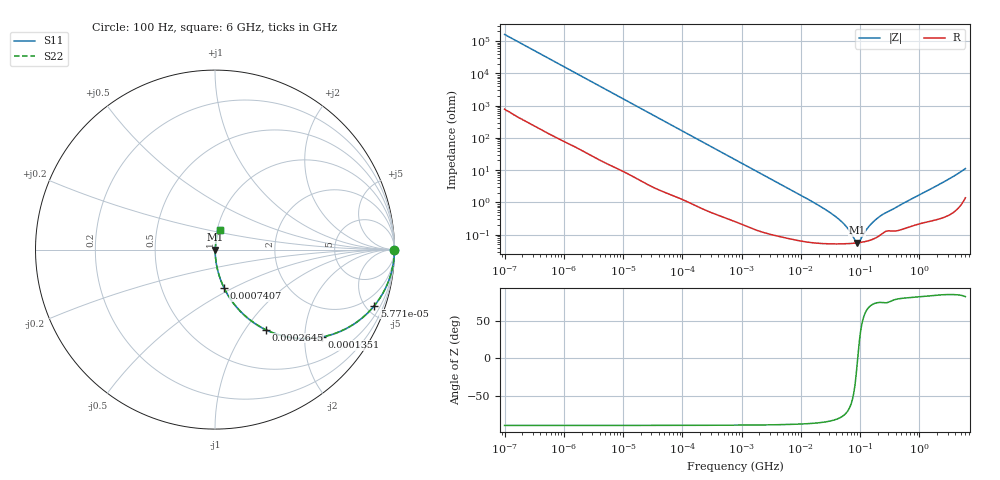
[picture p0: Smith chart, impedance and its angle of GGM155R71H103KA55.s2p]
!Murata Part Number: GGM155R71H103KA55
!These Parameters are Measured in Series Mode Connection
!Data Generated on Jun 19, 2026
!  o--ll--o
!Port1  Port2
!  o------o
!Operation Temp=25[degC], DC Bias Voltage=0[V]
!Freq. Start=100[Hz] Stop=6[GHz] 401[Steps]
# Hz S RI R 50
!Freq.(Hz) S11(Real) S11(Imag) S21(Real) S21(Imag) S12(Real) S12(Imag) S22(Real) S22(Imag)
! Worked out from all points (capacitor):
!   401 points, 100 Hz to 6 GHz, reference 50 ohm
!   read as one part in series: C = 9.88 nF near 109 Hz
!   lowest |Z| = 56.2 mohm at 89.18 MHz (marker M1)
!   series resonance near 91.21 MHz, so ESL is about 310 pH
!   S11 on the Smith chart (normalised r, x): 100 Hz: open; 57.71 kHz: 1.04, -5.69; 135.1 kHz: 1.02, -2.44; 264.5 kHz: 1.01, -1.25; 740.7 kHz: 1.01, -0.45; 6 GHz: 1.03, +0.22
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100  1 -0.000622  3.4e-06 0.000622  3.4e-06 0.000622  1 -0.000622
2008  0.9998 -0.0124  0.000216 0.0124  0.000216 0.0124  0.9998 -0.0124
12041  0.9942 -0.0733  0.00583 0.0733  0.00583 0.0733  0.9942 -0.0733
40335  0.9416 -0.2314  0.0584 0.2314  0.0584 0.2314  0.9416 -0.2314
57709  0.8883 -0.3117  0.1117 0.3117  0.1117 0.3117  0.8883 -0.3117
135116  0.5971 -0.4866  0.4029 0.4866  0.4029 0.4866  0.5971 -0.4866
264476  0.2825 -0.4459  0.7175 0.4459  0.7175 0.4459  0.2825 -0.4459
432798  0.1302 -0.3316  0.8698 0.3316  0.8698 0.3316  0.1302 -0.3316
740679  0.0502 -0.2126  0.9498 0.2126  0.9498 0.2126  0.0502 -0.2126
774597  0.0462 -0.2042  0.9538 0.2042  0.9538 0.2042  0.0462 -0.2042
2594782  0.00524 -0.0641  0.9948 0.0641  0.9948 0.0641  0.00524 -0.0641
1.555665e7  0.000675 -0.0106  0.9993 0.0106  0.9993 0.0106  0.000675 -0.0106
4.556224e7  0.000525 -0.0028  0.9995 0.0028  0.9995 0.0028  0.000525 -0.0028
5.960426e7  0.000527 -0.00163  0.9995 0.00163  0.9995 0.00163  0.000527 -0.00163
8.154455e7  0.000546 -0.000417  0.9995 0.000417  0.9995 0.000417  0.000546 -0.000417
8.918374e7  0.000556 -8.28e-05  0.9994 8.28e-05  0.9994 8.28e-05  0.000556 -8.28e-05
9.753859e7  0.000568 0.000251  0.9994 -0.000251  0.9994 -0.000251  0.000568 0.000251
1.334425e8  0.000638 0.00145  0.9994 -0.00145  0.9994 -0.00145  0.000638 0.00145
1.669249e8  0.000736 0.00238  0.9993 -0.00238  0.9993 -0.00238  0.000736 0.00238
3.124326e8  0.00134 0.00521  0.9987 -0.00521  0.9987 -0.00521  0.00134 0.00521
2.048624e9  0.00411 0.0338  0.9959 -0.0338  0.9959 -0.0338  0.00411 0.0338
6e9  0.0254 0.1071  0.9746 -0.1071  0.9746 -0.1071  0.0254 0.1071
